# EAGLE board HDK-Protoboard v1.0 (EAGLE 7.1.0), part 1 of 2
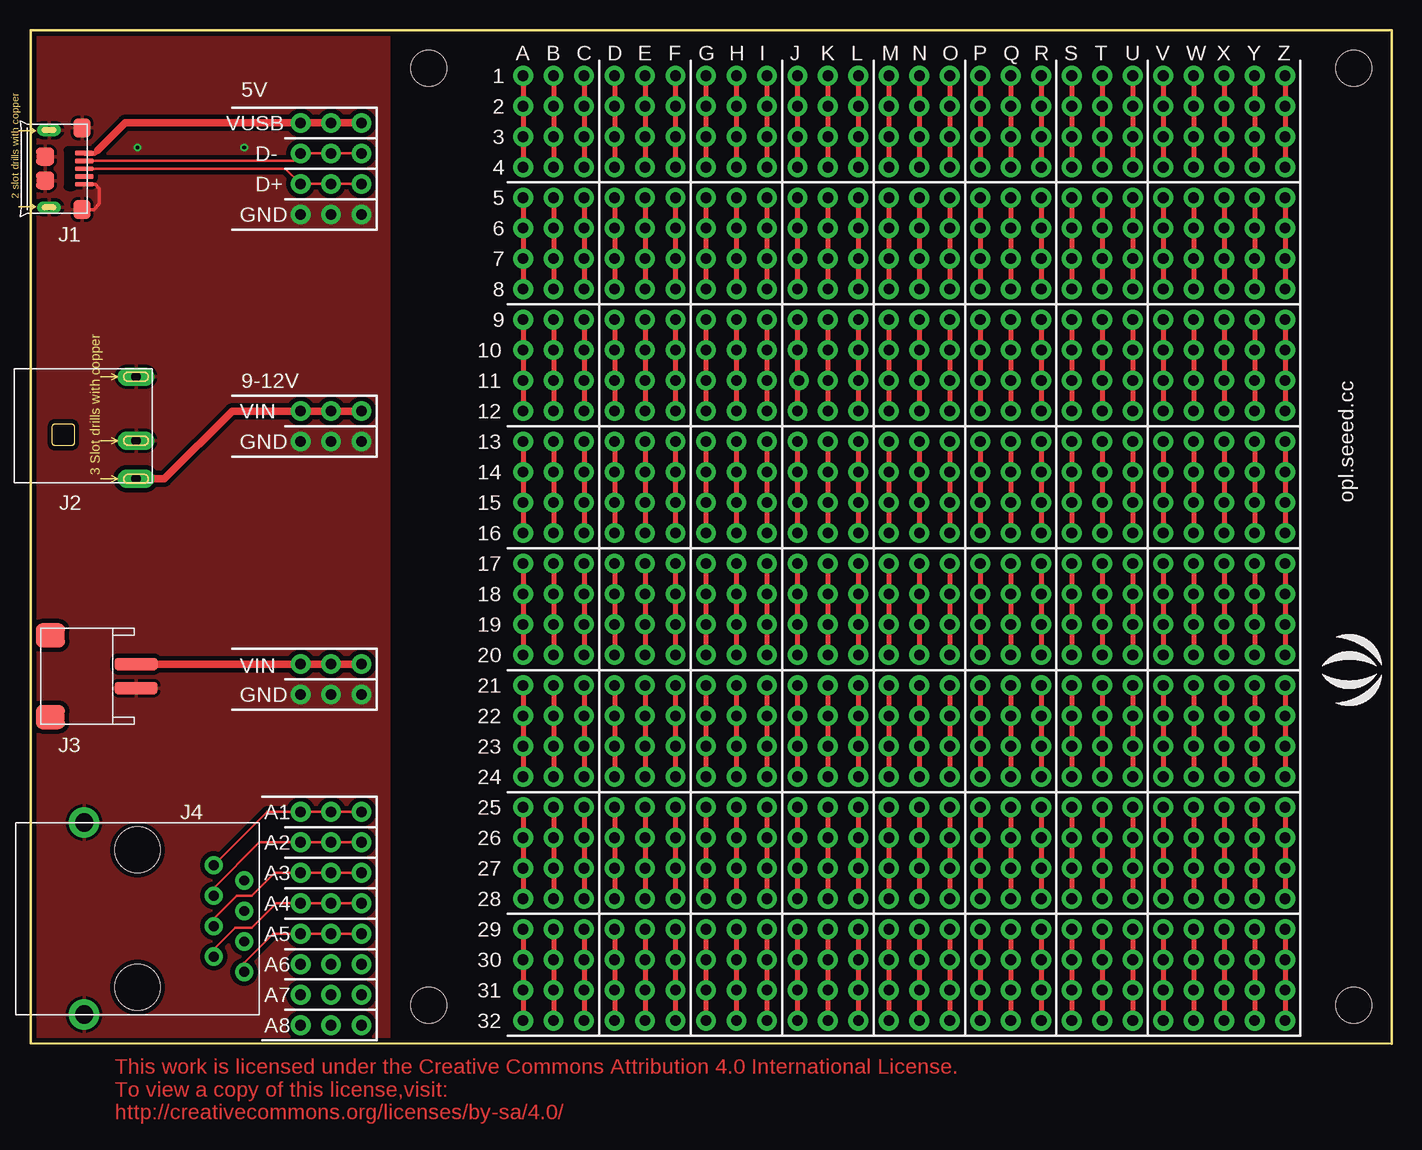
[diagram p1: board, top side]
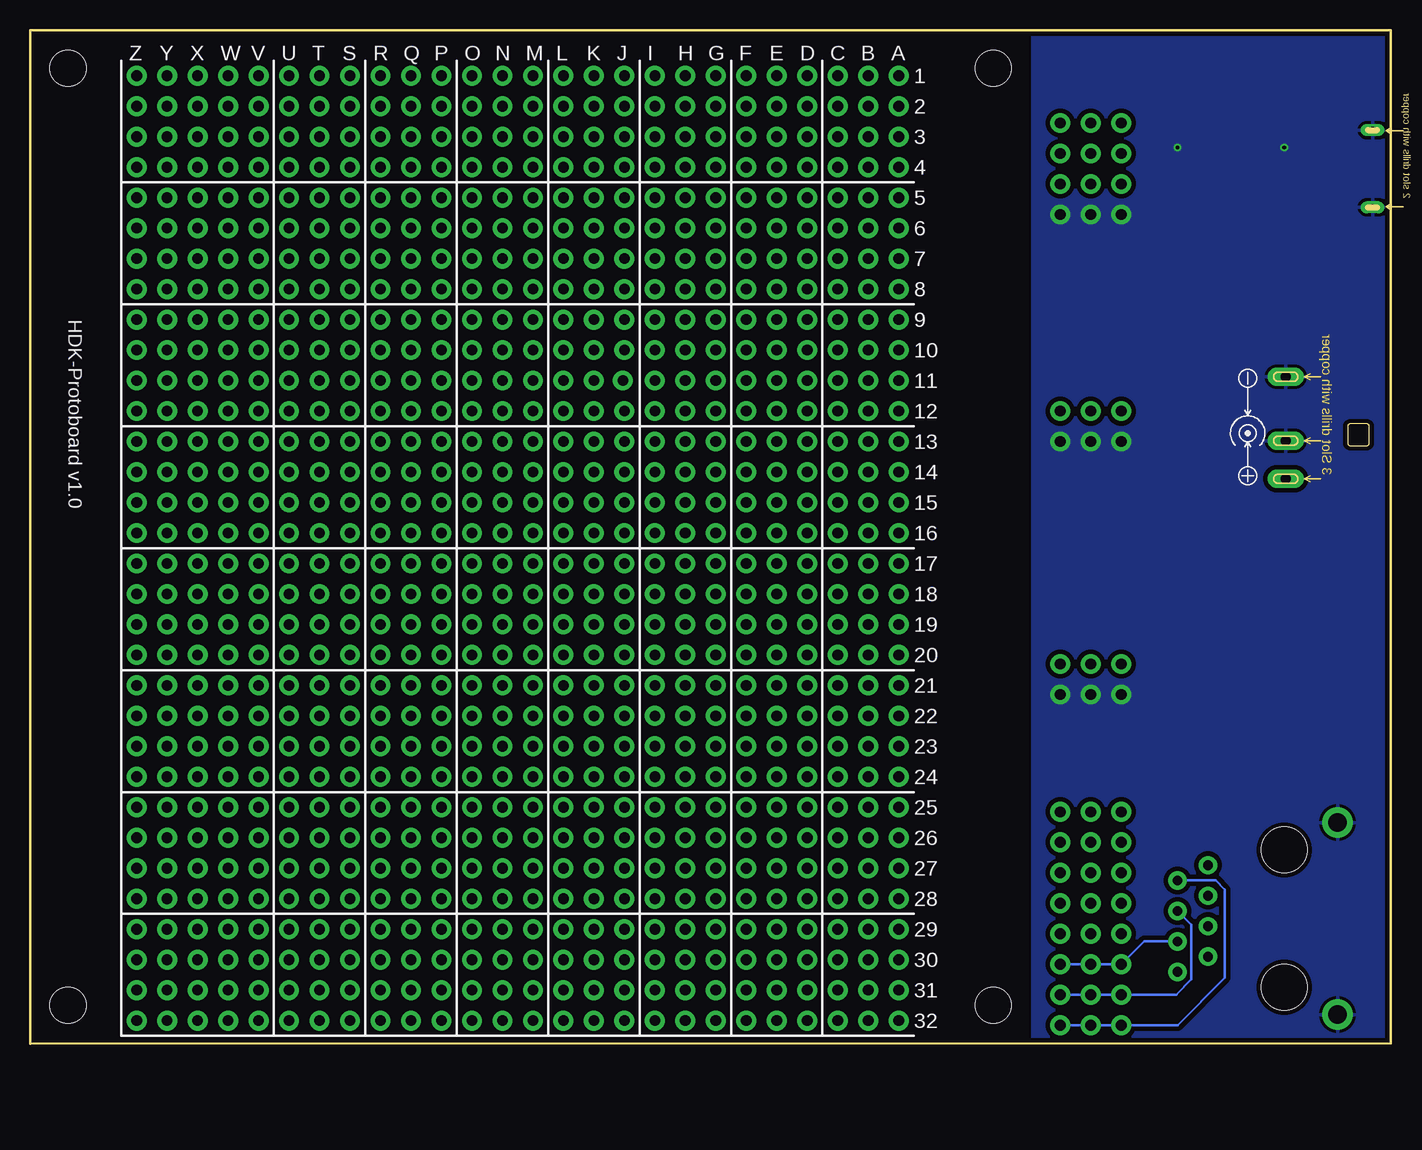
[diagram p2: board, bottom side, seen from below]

Size 113.41 x 84.46 mm. Coordinates in mm from the lower left corner, seen from the top.
Outline: 113.41,0 113.41,84.45 0,84.46 0,0.01 113.41,0
Copper layers (1*16): Top 0.035mm / dielectric 1.5mm / Bottom 0.035mm
Design rules "SeeedStudio_2layer_DRU_no_angle_20140221 *": minimum track width 1mil, minimum drill 12mil, track to track 6mil, track to pad 6mil, pad to pad 6mil, via to via 6mil, smd to smd 0mil, copper to edge 10mil, drill to drill 10mil, minimum pad ring 10mil, minimum via ring 6mil, stop-mask expansion 2mil, vias tented up to drill 25mil, thermal gap 10mil
Net classes: 2 gnd: width 0.305 mm, drill 0.559 mm, clearance 0.254 mm; 3 none3: width 0.203 mm, drill 0.305 mm, clearance 0.203 mm; 4 aref: width 0.406 mm, drill 0.61 mm, clearance 0.254 mm
Holes 3 mm at 110.24,81.28 110.24,3.18 33.15,81.28 33.15,3.18

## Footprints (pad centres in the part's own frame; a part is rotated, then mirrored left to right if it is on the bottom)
MICRO-USB5+4P-SMD-0.65-B-NO-HOLE = smd 0.381 x 1.524: 1 -1.3,-0.25; 2 -0.65,-0.25; 3 0,-0.25; 4 0.65,-0.25; 5 1.3,-0.25 | smd 1.6 x 1.397: S1 -3.4,-0.427; S6 3.4,-0.427 | drill 0.508 pad 1.016 long: S2 -3.226,-3.175; S5 3.226,-3.175 | smd 1.5 x 1.5: S3 -1,-3.5; S4 1,-3.5
DCJ3P-11.6X9.6X7.0MM = drill 0.813 pad 1.524 long: + 4.381,10.16; - -4.128,10.16; CDN 1.206,10.16
HW2-SMD-2.0-90D = smd 2 x 2.4: 3 3.4,-2.181; 4 -3.4,-2.181 | smd 1 x 3.6: + -1,4.953; - 1,4.953
RJ45-8P-20.4X16MM = drill 0.813 pad 1.524: A1 -2.54,5.08; A2 -2.54,2.54; A3 -2.54,0; A4 -2.54,-2.54; A5 0,-3.81; A6 0,-1.27; A7 0,1.27; A8 0,3.81 | drill 1.524 pad 2.54: GND0 -13.335,8.636; GND1 -13.335,-7.366 | hole 3.81: -8.89,-5.08; -8.89,6.35

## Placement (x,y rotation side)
FR1  [SEEEDSTUDIO-PCB-FRAME]  not placed on the board
J1  [MICRO-USB5+4P-SMD-0.65-B-NO-HOLE]  4.7,72.9 270 top
J2  [DCJ3P-11.6X9.6X7.0MM]  -1.4,51.44 270 top
J3  [HW2-SMD-2.0-90D]  3.81,30.61 270 top
J4  CONNECTER_RJ45_X1_DD  [RJ45-8P-20.4X16MM]  17.78,9.78 0 top
U$2  [SEEED-SILK-280*268MIL]  110.87,31.12 90 top

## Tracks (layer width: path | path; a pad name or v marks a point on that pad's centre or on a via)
A1  (via drill 0.89 pad 1.65)
  Top 0.203: J4.A1 19.69,19.31 v22.48,19.31 27.56,19.31
A2  (via drill 0.89 pad 1.65)
  Top 0.203: J4.A2 15.24,12.96 19.05,16.77 v22.48,16.77 27.56,16.77
A3  (via drill 0.89 pad 1.65)
  Top 0.203: J4.A3 15.24,10.42 17.14,12.32 18.41,12.32 20.32,14.23 v22.48,14.23 27.56,14.23
A4  (via drill 0.89 pad 1.65)
  Top 0.203: J4.A4 15.24,7.88 17.02,9.65 18.41,9.65 20.45,11.69 v22.48,11.69 27.56,11.69
A5  (via drill 0.89 pad 1.65)
  Top 0.203: J4.A5 17.78,6.73 20.19,9.15 v22.48,9.15 27.56,9.15
A6  (via drill 0.89 pad 1.65)
  Bottom 0.203: J4.A6 20.57,8.51 v22.48,6.61 27.56,6.61
A7  (via drill 0.89 pad 1.65)
  Bottom 0.203: J4.A7 16.64,9.91 16.64,5.34 17.91,4.07 v22.48,4.07 27.56,4.07
A8  (via drill 0.89 pad 1.65)
  Bottom 0.203: J4.A8 14.61,13.59 13.84,12.83 13.84,5.46 17.78,1.53 v22.48,1.53 27.56,1.53
D+2  (via drill 0.89 pad 1.65)
  Top 0.203: J1.3 21.21,72.9 v22.48,71.63 v25.02,71.63 v27.56,71.63
D-2  (via drill 0.89 pad 1.65)
  Top 0.203: J1.2 21.86,73.55 v22.48,74.17 v25.02,74.17 v27.56,74.17
GND  (via drill 0.3 pad 0.64, 0.89 pad 1.65)
  Top 0.305: J1.5 5.36,71.6 5.72,71.25 5.72,69.98 5.24,69.5 J1.S6
  other vias: 22.48,29.09 25.02,29.09 27.56,29.09 22.48,50.17 25.02,50.17 27.56,50.17 22.48,69.09 25.02,69.09 27.56,69.09 8.89,74.68 17.78,74.68
  pour Bottom (isolate 0.381, rank 6): -0.63,0 29.84,0 29.84,84.46 -0.63,84.46
  pour Top (isolate 0.381, rank 6): -0.63,0 29.84,0 29.84,84.46 -0.63,84.46
N$1  (via drill 0.89 pad 1.65)
  other vias: 41.02,1.91
N$2  (via drill 0.89 pad 1.65)
  other vias: 43.56,1.91
N$3  (via drill 0.89 pad 1.65)
  other vias: 46.1,1.91
N$4  (via drill 0.89 pad 1.65)
  other vias: 48.64,1.91
N$5  (via drill 0.89 pad 1.65)
  other vias: 51.18,1.91
N$6  (via drill 0.89 pad 1.65)
  other vias: 41.02,4.45
N$7  (via drill 0.89 pad 1.65)
  other vias: 43.56,4.45
N$8  (via drill 0.89 pad 1.65)
  other vias: 46.1,4.45
N$9  (via drill 0.89 pad 1.65)
  other vias: 48.64,4.45
N$10  (via drill 0.89 pad 1.65)
  other vias: 51.18,4.45
N$11  (via drill 0.89 pad 1.65)
  other vias: 53.72,1.91
N$12  (via drill 0.89 pad 1.65)
  other vias: 53.72,4.45
N$13  (via drill 0.89 pad 1.65)
  other vias: 56.26,4.45
N$14  (via drill 0.89 pad 1.65)
  other vias: 56.26,1.91
N$15  (via drill 0.89 pad 1.65)
  other vias: 58.8,4.45
N$16  (via drill 0.89 pad 1.65)
  other vias: 58.8,1.91
N$18  (via drill 0.89 pad 1.65)
  other vias: 61.34,4.45
N$19  (via drill 0.89 pad 1.65)
  other vias: 66.42,1.91
N$20  (via drill 0.89 pad 1.65)
  other vias: 68.96,4.45
N$21  (via drill 0.89 pad 1.65)
  other vias: 68.96,1.91
N$22  (via drill 0.89 pad 1.65)
  other vias: 71.5,4.45
N$23  (via drill 0.89 pad 1.65)
  other vias: 71.5,1.91
N$24  (via drill 0.89 pad 1.65)
  other vias: 74.04,4.45
N$25  (via drill 0.89 pad 1.65)
  other vias: 74.04,1.91
N$26  (via drill 0.89 pad 1.65)
  other vias: 76.58,4.45
N$27  (via drill 0.89 pad 1.65)
  other vias: 76.58,1.91
N$28  (via drill 0.89 pad 1.65)
  other vias: 79.12,4.45
N$29  (via drill 0.89 pad 1.65)
  other vias: 79.12,1.91
N$30  (via drill 0.89 pad 1.65)
  other vias: 81.66,4.45
N$31  (via drill 0.89 pad 1.65)
  other vias: 81.66,1.91
N$32  (via drill 0.89 pad 1.65)
  other vias: 84.2,4.45
N$33  (via drill 0.89 pad 1.65)
  other vias: 84.2,1.91
N$34  (via drill 0.89 pad 1.65)
  other vias: 86.74,1.91
N$35  (via drill 0.89 pad 1.65)
  other vias: 89.28,1.91
N$36  (via drill 0.89 pad 1.65)
  other vias: 91.82,1.91
N$37  (via drill 0.89 pad 1.65)
  other vias: 94.36,1.91
N$38  (via drill 0.89 pad 1.65)
  other vias: 96.9,1.91
N$39  (via drill 0.89 pad 1.65)
  other vias: 99.44,1.91
N$40  (via drill 0.89 pad 1.65)
  other vias: 101.98,1.91
N$41  (via drill 0.89 pad 1.65)
  other vias: 104.52,1.91
N$42  (via drill 0.89 pad 1.65)
  other vias: 86.74,4.45
N$43  (via drill 0.89 pad 1.65)
  other vias: 89.28,4.45
N$44  (via drill 0.89 pad 1.65)
  other vias: 91.82,4.45
N$45  (via drill 0.89 pad 1.65)
  other vias: 94.36,4.45
N$46  (via drill 0.89 pad 1.65)
  other vias: 96.9,4.45
N$47  (via drill 0.89 pad 1.65)
  other vias: 99.44,4.45
N$48  (via drill 0.89 pad 1.65)
  other vias: 101.98,4.45
N$49  (via drill 0.89 pad 1.65)
  other vias: 104.52,4.45
N$50  (via drill 0.89 pad 1.65)
  other vias: 41.02,6.99
N$51  (via drill 0.89 pad 1.65)
  other vias: 43.56,6.99
N$52  (via drill 0.89 pad 1.65)
  other vias: 46.1,6.99
N$53  (via drill 0.89 pad 1.65)
  other vias: 48.64,6.99
N$54  (via drill 0.89 pad 1.65)
  other vias: 51.18,6.99
N$55  (via drill 0.89 pad 1.65)
  Top 0.406: v41.02,9.53 41.02,1.91
N$56  (via drill 0.89 pad 1.65)
  other vias: 43.56,9.53
N$57  (via drill 0.89 pad 1.65)
  other vias: 46.1,9.53
N$58  (via drill 0.89 pad 1.65)
  other vias: 48.64,9.53
N$59  (via drill 0.89 pad 1.65)
  other vias: 51.18,9.53
N$60  (via drill 0.89 pad 1.65)
  other vias: 53.72,6.99
N$61  (via drill 0.89 pad 1.65)
  other vias: 53.72,9.53
N$62  (via drill 0.89 pad 1.65)
  other vias: 56.26,9.53
N$63  (via drill 0.89 pad 1.65)
  other vias: 56.26,6.99
N$64  (via drill 0.89 pad 1.65)
  other vias: 58.8,9.53
N$65  (via drill 0.89 pad 1.65)
  other vias: 58.8,6.99
N$67  (via drill 0.89 pad 1.65)
  other vias: 61.34,9.53
N$68  (via drill 0.89 pad 1.65)
  other vias: 66.42,6.99
N$69  (via drill 0.89 pad 1.65)
  other vias: 68.96,9.53
N$70  (via drill 0.89 pad 1.65)
  other vias: 68.96,6.99
N$71  (via drill 0.89 pad 1.65)
  other vias: 71.5,9.53
N$72  (via drill 0.89 pad 1.65)
  other vias: 71.5,6.99
N$73  (via drill 0.89 pad 1.65)
  other vias: 74.04,9.53
N$74  (via drill 0.89 pad 1.65)
  other vias: 74.04,6.99
N$75  (via drill 0.89 pad 1.65)
  other vias: 76.58,9.53
N$76  (via drill 0.89 pad 1.65)
  other vias: 76.58,6.99
N$77  (via drill 0.89 pad 1.65)
  other vias: 79.12,9.53
N$78  (via drill 0.89 pad 1.65)
  other vias: 79.12,6.99
N$79  (via drill 0.89 pad 1.65)
  other vias: 81.66,9.53
N$80  (via drill 0.89 pad 1.65)
  other vias: 81.66,6.99
N$81  (via drill 0.89 pad 1.65)
  other vias: 84.2,9.53
N$82  (via drill 0.89 pad 1.65)
  other vias: 84.2,6.99
N$83  (via drill 0.89 pad 1.65)
  other vias: 86.74,6.99
N$84  (via drill 0.89 pad 1.65)
  other vias: 89.28,6.99
N$85  (via drill 0.89 pad 1.65)
  other vias: 91.82,6.99
N$86  (via drill 0.89 pad 1.65)
  other vias: 94.36,6.99
N$87  (via drill 0.89 pad 1.65)
  other vias: 96.9,6.99
N$88  (via drill 0.89 pad 1.65)
  other vias: 99.44,6.99
N$89  (via drill 0.89 pad 1.65)
  other vias: 101.98,6.99
N$90  (via drill 0.89 pad 1.65)
  other vias: 104.52,6.99
N$91  (via drill 0.89 pad 1.65)
  other vias: 86.74,9.53
N$92  (via drill 0.89 pad 1.65)
  other vias: 89.28,9.53
N$93  (via drill 0.89 pad 1.65)
  other vias: 91.82,9.53
N$94  (via drill 0.89 pad 1.65)
  other vias: 94.36,9.53
N$95  (via drill 0.89 pad 1.65)
  other vias: 96.9,9.53
N$96  (via drill 0.89 pad 1.65)
  other vias: 99.44,9.53
N$97  (via drill 0.89 pad 1.65)
  other vias: 101.98,9.53
N$98  (via drill 0.89 pad 1.65)
  other vias: 104.52,9.53
N$99  (via drill 0.89 pad 1.65)
  other vias: 41.02,12.07
N$100  (via drill 0.89 pad 1.65)
  other vias: 43.56,12.07
N$101  (via drill 0.89 pad 1.65)
  other vias: 46.1,12.07
N$102  (via drill 0.89 pad 1.65)
  other vias: 48.64,12.07
N$103  (via drill 0.89 pad 1.65)
  other vias: 51.18,12.07
N$104  (via drill 0.89 pad 1.65)
  other vias: 41.02,14.61
N$105  (via drill 0.89 pad 1.65)
  other vias: 43.56,14.61
N$106  (via drill 0.89 pad 1.65)
  other vias: 46.1,14.61
N$107  (via drill 0.89 pad 1.65)
  other vias: 48.64,14.61
N$108  (via drill 0.89 pad 1.65)
  other vias: 51.18,14.61
N$109  (via drill 0.89 pad 1.65)
  other vias: 53.72,12.07
N$110  (via drill 0.89 pad 1.65)
  other vias: 53.72,14.61
N$111  (via drill 0.89 pad 1.65)
  other vias: 56.26,14.61
N$112  (via drill 0.89 pad 1.65)
  other vias: 56.26,12.07
N$113  (via drill 0.89 pad 1.65)
  other vias: 58.8,14.61
N$114  (via drill 0.89 pad 1.65)
  other vias: 58.8,12.07
N$116  (via drill 0.89 pad 1.65)
  other vias: 61.34,14.61
N$117  (via drill 0.89 pad 1.65)
  other vias: 66.42,12.07
N$118  (via drill 0.89 pad 1.65)
  other vias: 68.96,14.61
N$119  (via drill 0.89 pad 1.65)
  other vias: 68.96,12.07
N$120  (via drill 0.89 pad 1.65)
  other vias: 71.5,14.61
N$121  (via drill 0.89 pad 1.65)
  other vias: 71.5,12.07
N$122  (via drill 0.89 pad 1.65)
  other vias: 74.04,14.61
N$123  (via drill 0.89 pad 1.65)
  other vias: 74.04,12.07
N$124  (via drill 0.89 pad 1.65)
  other vias: 76.58,14.61
N$125  (via drill 0.89 pad 1.65)
  other vias: 76.58,12.07
N$126  (via drill 0.89 pad 1.65)
  other vias: 79.12,14.61
N$127  (via drill 0.89 pad 1.65)
  other vias: 79.12,12.07
N$128  (via drill 0.89 pad 1.65)
  other vias: 81.66,14.61
N$129  (via drill 0.89 pad 1.65)
  other vias: 81.66,12.07
N$130  (via drill 0.89 pad 1.65)
  other vias: 84.2,14.61
N$131  (via drill 0.89 pad 1.65)
  other vias: 84.2,12.07
N$132  (via drill 0.89 pad 1.65)
  other vias: 86.74,12.07
N$133  (via drill 0.89 pad 1.65)
  other vias: 89.28,12.07
N$134  (via drill 0.89 pad 1.65)
  other vias: 91.82,12.07
N$135  (via drill 0.89 pad 1.65)
  other vias: 94.36,12.07
N$136  (via drill 0.89 pad 1.65)
  other vias: 96.9,12.07
N$137  (via drill 0.89 pad 1.65)
  other vias: 99.44,12.07
N$138  (via drill 0.89 pad 1.65)
  other vias: 101.98,12.07
N$139  (via drill 0.89 pad 1.65)
  other vias: 104.52,12.07
N$140  (via drill 0.89 pad 1.65)
  other vias: 86.74,14.61
N$141  (via drill 0.89 pad 1.65)
  other vias: 89.28,14.61
N$142  (via drill 0.89 pad 1.65)
  other vias: 91.82,14.61
N$143  (via drill 0.89 pad 1.65)
  other vias: 94.36,14.61
N$144  (via drill 0.89 pad 1.65)
  other vias: 96.9,14.61
N$145  (via drill 0.89 pad 1.65)
  other vias: 99.44,14.61
N$146  (via drill 0.89 pad 1.65)
  other vias: 101.98,14.61
N$147  (via drill 0.89 pad 1.65)
  other vias: 104.52,14.61
N$148  (via drill 0.89 pad 1.65)
  other vias: 41.02,17.15
N$149  (via drill 0.89 pad 1.65)
  other vias: 43.56,17.15
N$150  (via drill 0.89 pad 1.65)
  other vias: 46.1,17.15
N$151  (via drill 0.89 pad 1.65)
  other vias: 48.64,17.15
N$152  (via drill 0.89 pad 1.65)
  other vias: 51.18,17.15
N$153  (via drill 0.89 pad 1.65)
  Top 0.406: v41.02,19.69 41.02,12.07
N$154  (via drill 0.89 pad 1.65)
  other vias: 43.56,19.69
N$155  (via drill 0.89 pad 1.65)
  other vias: 46.1,19.69
N$156  (via drill 0.89 pad 1.65)
  other vias: 48.64,19.69
N$157  (via drill 0.89 pad 1.65)
  other vias: 51.18,19.69
N$158  (via drill 0.89 pad 1.65)
  other vias: 53.72,17.15
N$159  (via drill 0.89 pad 1.65)
  other vias: 53.72,19.69
N$160  (via drill 0.89 pad 1.65)
  other vias: 56.26,19.69
N$161  (via drill 0.89 pad 1.65)
  other vias: 56.26,17.15
N$162  (via drill 0.89 pad 1.65)
  other vias: 58.8,19.69
N$163  (via drill 0.89 pad 1.65)
  other vias: 58.8,17.15
N$165  (via drill 0.89 pad 1.65)
  other vias: 61.34,19.69
N$166  (via drill 0.89 pad 1.65)
  other vias: 66.42,17.15
N$167  (via drill 0.89 pad 1.65)
  other vias: 68.96,19.69
N$168  (via drill 0.89 pad 1.65)
  other vias: 68.96,17.15
N$169  (via drill 0.89 pad 1.65)
  other vias: 71.5,19.69
N$170  (via drill 0.89 pad 1.65)
  other vias: 71.5,17.15
N$171  (via drill 0.89 pad 1.65)
  other vias: 74.04,19.69
N$172  (via drill 0.89 pad 1.65)
  other vias: 74.04,17.15
N$173  (via drill 0.89 pad 1.65)
  other vias: 76.58,19.69
N$174  (via drill 0.89 pad 1.65)
  other vias: 76.58,17.15
N$175  (via drill 0.89 pad 1.65)
  other vias: 79.12,19.69
N$176  (via drill 0.89 pad 1.65)
  other vias: 79.12,17.15
N$177  (via drill 0.89 pad 1.65)
  other vias: 81.66,19.69
N$178  (via drill 0.89 pad 1.65)
  other vias: 81.66,17.15
N$179  (via drill 0.89 pad 1.65)
  other vias: 84.2,19.69
N$180  (via drill 0.89 pad 1.65)
  other vias: 84.2,17.15
N$181  (via drill 0.89 pad 1.65)
  other vias: 86.74,17.15
N$182  (via drill 0.89 pad 1.65)
  other vias: 89.28,17.15
N$183  (via drill 0.89 pad 1.65)
  other vias: 91.82,17.15
N$184  (via drill 0.89 pad 1.65)
  other vias: 94.36,17.15
N$185  (via drill 0.89 pad 1.65)
  other vias: 96.9,17.15
N$186  (via drill 0.89 pad 1.65)
  other vias: 99.44,17.15
N$187  (via drill 0.89 pad 1.65)
  other vias: 101.98,17.15
N$188  (via drill 0.89 pad 1.65)
  other vias: 104.52,17.15
N$189  (via drill 0.89 pad 1.65)
  other vias: 86.74,19.69
N$190  (via drill 0.89 pad 1.65)
  other vias: 89.28,19.69
N$191  (via drill 0.89 pad 1.65)
  other vias: 91.82,19.69
N$192  (via drill 0.89 pad 1.65)
  other vias: 94.36,19.69
N$193  (via drill 0.89 pad 1.65)
  other vias: 96.9,19.69
N$194  (via drill 0.89 pad 1.65)
  other vias: 99.44,19.69
N$195  (via drill 0.89 pad 1.65)
  other vias: 101.98,19.69
N$196  (via drill 0.89 pad 1.65)
  other vias: 104.52,19.69
N$197  (via drill 0.89 pad 1.65)
  other vias: 41.02,22.23
N$198  (via drill 0.89 pad 1.65)
  other vias: 43.56,22.23
N$199  (via drill 0.89 pad 1.65)
  other vias: 46.1,22.23
N$200  (via drill 0.89 pad 1.65)
  other vias: 48.64,22.23
N$201  (via drill 0.89 pad 1.65)
  other vias: 51.18,22.23
N$202  (via drill 0.89 pad 1.65)
  other vias: 41.02,24.77
N$203  (via drill 0.89 pad 1.65)
  other vias: 43.56,24.77
N$204  (via drill 0.89 pad 1.65)
  other vias: 46.1,24.77
N$205  (via drill 0.89 pad 1.65)
  other vias: 48.64,24.77
N$206  (via drill 0.89 pad 1.65)
  other vias: 51.18,24.77
N$207  (via drill 0.89 pad 1.65)
  other vias: 53.72,22.23
N$208  (via drill 0.89 pad 1.65)
  other vias: 53.72,24.77
N$209  (via drill 0.89 pad 1.65)
  other vias: 56.26,24.77
N$210  (via drill 0.89 pad 1.65)
  other vias: 56.26,22.23
N$211  (via drill 0.89 pad 1.65)
  other vias: 58.8,24.77
N$212  (via drill 0.89 pad 1.65)
  other vias: 58.8,22.23
N$214  (via drill 0.89 pad 1.65)
  other vias: 61.34,24.77
N$215  (via drill 0.89 pad 1.65)
  other vias: 66.42,22.23
N$216  (via drill 0.89 pad 1.65)
  other vias: 68.96,24.77
N$217  (via drill 0.89 pad 1.65)
  other vias: 68.96,22.23
N$218  (via drill 0.89 pad 1.65)
  other vias: 71.5,24.77
N$219  (via drill 0.89 pad 1.65)
  other vias: 71.5,22.23
N$220  (via drill 0.89 pad 1.65)
  other vias: 74.04,24.77
N$221  (via drill 0.89 pad 1.65)
  other vias: 74.04,22.23
N$222  (via drill 0.89 pad 1.65)
  other vias: 76.58,24.77
N$223  (via drill 0.89 pad 1.65)
  other vias: 76.58,22.23
N$224  (via drill 0.89 pad 1.65)
  other vias: 79.12,24.77
N$225  (via drill 0.89 pad 1.65)
  other vias: 79.12,22.23
N$226  (via drill 0.89 pad 1.65)
  other vias: 81.66,24.77
N$227  (via drill 0.89 pad 1.65)
  other vias: 81.66,22.23
N$228  (via drill 0.89 pad 1.65)
  other vias: 84.2,24.77
N$229  (via drill 0.89 pad 1.65)
  other vias: 84.2,22.23
N$230  (via drill 0.89 pad 1.65)
  other vias: 86.74,22.23
N$231  (via drill 0.89 pad 1.65)
  other vias: 89.28,22.23
N$232  (via drill 0.89 pad 1.65)
  other vias: 91.82,22.23
N$233  (via drill 0.89 pad 1.65)
  other vias: 94.36,22.23
N$234  (via drill 0.89 pad 1.65)
  other vias: 96.9,22.23
N$235  (via drill 0.89 pad 1.65)
  other vias: 99.44,22.23
N$236  (via drill 0.89 pad 1.65)
  other vias: 101.98,22.23
N$237  (via drill 0.89 pad 1.65)
  other vias: 104.52,22.23
N$238  (via drill 0.89 pad 1.65)
  other vias: 86.74,24.77
N$239  (via drill 0.89 pad 1.65)
  other vias: 89.28,24.77
N$240  (via drill 0.89 pad 1.65)
  other vias: 91.82,24.77
N$241  (via drill 0.89 pad 1.65)
  other vias: 94.36,24.77
N$242  (via drill 0.89 pad 1.65)
  other vias: 96.9,24.77
N$243  (via drill 0.89 pad 1.65)
  other vias: 99.44,24.77
N$244  (via drill 0.89 pad 1.65)
  other vias: 101.98,24.77
N$245  (via drill 0.89 pad 1.65)
  other vias: 104.52,24.77
N$246  (via drill 0.89 pad 1.65)
  other vias: 41.02,27.31
N$247  (via drill 0.89 pad 1.65)
  other vias: 43.56,27.31
N$248  (via drill 0.89 pad 1.65)
  other vias: 46.1,27.31
N$249  (via drill 0.89 pad 1.65)
  other vias: 48.64,27.31
N$250  (via drill 0.89 pad 1.65)
  other vias: 51.18,27.31
N$251  (via drill 0.89 pad 1.65)
  Top 0.406: v41.02,29.85 41.02,22.23
N$252  (via drill 0.89 pad 1.65)
  other vias: 43.56,29.85
N$253  (via drill 0.89 pad 1.65)
  other vias: 46.1,29.85
N$254  (via drill 0.89 pad 1.65)
  other vias: 48.64,29.85
N$255  (via drill 0.89 pad 1.65)
  other vias: 51.18,29.85
N$256  (via drill 0.89 pad 1.65)
  other vias: 53.72,27.31
N$257  (via drill 0.89 pad 1.65)
  other vias: 53.72,29.85
N$258  (via drill 0.89 pad 1.65)
  other vias: 56.26,29.85
N$259  (via drill 0.89 pad 1.65)
  other vias: 56.26,27.31
N$260  (via drill 0.89 pad 1.65)
  other vias: 58.8,29.85
N$261  (via drill 0.89 pad 1.65)
  other vias: 58.8,27.31
N$263  (via drill 0.89 pad 1.65)
  other vias: 61.34,29.85
N$264  (via drill 0.89 pad 1.65)
  other vias: 66.42,27.31
N$265  (via drill 0.89 pad 1.65)
  other vias: 68.96,29.85
N$266  (via drill 0.89 pad 1.65)
  other vias: 68.96,27.31
N$267  (via drill 0.89 pad 1.65)
  other vias: 71.5,29.85
N$268  (via drill 0.89 pad 1.65)
  other vias: 71.5,27.31
N$269  (via drill 0.89 pad 1.65)
  other vias: 74.04,29.85
N$270  (via drill 0.89 pad 1.65)
  other vias: 74.04,27.31
N$271  (via drill 0.89 pad 1.65)
  other vias: 76.58,29.85
N$272  (via drill 0.89 pad 1.65)
  other vias: 76.58,27.31
N$273  (via drill 0.89 pad 1.65)
  other vias: 79.12,29.85
N$274  (via drill 0.89 pad 1.65)
  other vias: 79.12,27.31
N$275  (via drill 0.89 pad 1.65)
  other vias: 81.66,29.85
N$276  (via drill 0.89 pad 1.65)
  other vias: 81.66,27.31
N$277  (via drill 0.89 pad 1.65)
  other vias: 84.2,29.85
N$278  (via drill 0.89 pad 1.65)
  other vias: 84.2,27.31
N$279  (via drill 0.89 pad 1.65)
  other vias: 86.74,27.31
N$280  (via drill 0.89 pad 1.65)
  other vias: 89.28,27.31
N$281  (via drill 0.89 pad 1.65)
  other vias: 91.82,27.31
N$282  (via drill 0.89 pad 1.65)
  other vias: 94.36,27.31
N$283  (via drill 0.89 pad 1.65)
  other vias: 96.9,27.31
N$284  (via drill 0.89 pad 1.65)
  other vias: 99.44,27.31
N$285  (via drill 0.89 pad 1.65)
  other vias: 101.98,27.31
N$286  (via drill 0.89 pad 1.65)
  other vias: 104.52,27.31
N$287  (via drill 0.89 pad 1.65)
  other vias: 86.74,29.85
N$288  (via drill 0.89 pad 1.65)
  other vias: 89.28,29.85
N$289  (via drill 0.89 pad 1.65)
  other vias: 91.82,29.85
N$290  (via drill 0.89 pad 1.65)
  other vias: 94.36,29.85
N$291  (via drill 0.89 pad 1.65)
  other vias: 96.9,29.85
N$292  (via drill 0.89 pad 1.65)
  other vias: 99.44,29.85
N$293  (via drill 0.89 pad 1.65)
  other vias: 101.98,29.85
N$294  (via drill 0.89 pad 1.65)
  other vias: 104.52,29.85
N$295  (via drill 0.89 pad 1.65)
  other vias: 41.02,32.39
N$296  (via drill 0.89 pad 1.65)
  other vias: 43.56,32.39
N$297  (via drill 0.89 pad 1.65)
  other vias: 46.1,32.39
N$298  (via drill 0.89 pad 1.65)
  other vias: 48.64,32.39
N$299  (via drill 0.89 pad 1.65)
  other vias: 51.18,32.39
N$300  (via drill 0.89 pad 1.65)
  other vias: 41.02,34.93
N$301  (via drill 0.89 pad 1.65)
  other vias: 43.56,34.93
N$302  (via drill 0.89 pad 1.65)
  other vias: 46.1,34.93
N$303  (via drill 0.89 pad 1.65)
  other vias: 48.64,34.93
N$304  (via drill 0.89 pad 1.65)
  other vias: 51.18,34.93
N$305  (via drill 0.89 pad 1.65)
  other vias: 53.72,32.39
N$306  (via drill 0.89 pad 1.65)
  other vias: 53.72,34.93
N$307  (via drill 0.89 pad 1.65)
  other vias: 56.26,34.93
N$308  (via drill 0.89 pad 1.65)
  other vias: 56.26,32.39
N$309  (via drill 0.89 pad 1.65)
  other vias: 58.8,34.93
N$310  (via drill 0.89 pad 1.65)
  other vias: 58.8,32.39
N$312  (via drill 0.89 pad 1.65)
  other vias: 61.34,34.93
N$313  (via drill 0.89 pad 1.65)
  other vias: 66.42,32.39
N$314  (via drill 0.89 pad 1.65)
  other vias: 68.96,34.93
N$315  (via drill 0.89 pad 1.65)
  other vias: 68.96,32.39
N$316  (via drill 0.89 pad 1.65)
  other vias: 71.5,34.93
N$317  (via drill 0.89 pad 1.65)
  other vias: 71.5,32.39
N$318  (via drill 0.89 pad 1.65)
  other vias: 74.04,34.93
N$319  (via drill 0.89 pad 1.65)
  other vias: 74.04,32.39
N$320  (via drill 0.89 pad 1.65)
  other vias: 76.58,34.93
N$321  (via drill 0.89 pad 1.65)
  other vias: 76.58,32.39
N$322  (via drill 0.89 pad 1.65)
  other vias: 79.12,34.93
N$323  (via drill 0.89 pad 1.65)
  other vias: 79.12,32.39
N$324  (via drill 0.89 pad 1.65)
  other vias: 81.66,34.93
N$325  (via drill 0.89 pad 1.65)
  other vias: 81.66,32.39
N$326  (via drill 0.89 pad 1.65)
  other vias: 84.2,34.93
N$327  (via drill 0.89 pad 1.65)
  other vias: 84.2,32.39
N$328  (via drill 0.89 pad 1.65)
  other vias: 86.74,32.39
N$329  (via drill 0.89 pad 1.65)
  other vias: 89.28,32.39
N$330  (via drill 0.89 pad 1.65)
  other vias: 91.82,32.39
N$331  (via drill 0.89 pad 1.65)
  other vias: 94.36,32.39
N$332  (via drill 0.89 pad 1.65)
  other vias: 96.9,32.39
N$333  (via drill 0.89 pad 1.65)
  other vias: 99.44,32.39
N$334  (via drill 0.89 pad 1.65)
  other vias: 101.98,32.39
N$335  (via drill 0.89 pad 1.65)
  other vias: 104.52,32.39
N$336  (via drill 0.89 pad 1.65)
  other vias: 86.74,34.93
N$337  (via drill 0.89 pad 1.65)
  other vias: 89.28,34.93
N$338  (via drill 0.89 pad 1.65)
  other vias: 91.82,34.93
N$339  (via drill 0.89 pad 1.65)
  other vias: 94.36,34.93
N$340  (via drill 0.89 pad 1.65)
  other vias: 96.9,34.93
N$341  (via drill 0.89 pad 1.65)
  other vias: 99.44,34.93
N$342  (via drill 0.89 pad 1.65)
  other vias: 101.98,34.93
N$343  (via drill 0.89 pad 1.65)
  other vias: 104.52,34.93
N$344  (via drill 0.89 pad 1.65)
  other vias: 41.02,37.47
N$345  (via drill 0.89 pad 1.65)
  other vias: 43.56,37.47
N$346  (via drill 0.89 pad 1.65)
  other vias: 46.1,37.47
N$347  (via drill 0.89 pad 1.65)
  other vias: 48.64,37.47
N$348  (via drill 0.89 pad 1.65)
  other vias: 51.18,37.47
N$349  (via drill 0.89 pad 1.65)
  Top 0.406: v41.02,40.01 41.02,32.39
N$350  (via drill 0.89 pad 1.65)
  other vias: 43.56,40.01
N$351  (via drill 0.89 pad 1.65)
  other vias: 46.1,40.01
N$352  (via drill 0.89 pad 1.65)
  other vias: 48.64,40.01
N$353  (via drill 0.89 pad 1.65)
  other vias: 51.18,40.01
N$354  (via drill 0.89 pad 1.65)
  other vias: 53.72,37.47
N$355  (via drill 0.89 pad 1.65)
  other vias: 53.72,40.01
N$356  (via drill 0.89 pad 1.65)
  other vias: 56.26,40.01
N$357  (via drill 0.89 pad 1.65)
  other vias: 56.26,37.47
N$358  (via drill 0.89 pad 1.65)
  other vias: 58.8,40.01
N$359  (via drill 0.89 pad 1.65)
  other vias: 58.8,37.47
N$360  (via drill 0.89 pad 1.65)
  other vias: 61.34,37.47
N$361  (via drill 0.89 pad 1.65)
  other vias: 61.34,40.01
N$362  (via drill 0.89 pad 1.65)
  other vias: 66.42,37.47
N$363  (via drill 0.89 pad 1.65)
  other vias: 68.96,40.01
N$364  (via drill 0.89 pad 1.65)
  other vias: 68.96,37.47
N$365  (via drill 0.89 pad 1.65)
  other vias: 71.5,40.01
N$366  (via drill 0.89 pad 1.65)
  other vias: 71.5,37.47
N$367  (via drill 0.89 pad 1.65)
  other vias: 74.04,40.01
N$368  (via drill 0.89 pad 1.65)
  other vias: 74.04,37.47
N$369  (via drill 0.89 pad 1.65)
  other vias: 76.58,40.01
N$370  (via drill 0.89 pad 1.65)
  other vias: 76.58,37.47
N$371  (via drill 0.89 pad 1.65)
  other vias: 79.12,40.01
N$372  (via drill 0.89 pad 1.65)
  other vias: 79.12,37.47
N$373  (via drill 0.89 pad 1.65)
  other vias: 81.66,40.01
N$374  (via drill 0.89 pad 1.65)
  other vias: 81.66,37.47
N$375  (via drill 0.89 pad 1.65)
  other vias: 84.2,40.01
N$376  (via drill 0.89 pad 1.65)
  other vias: 84.2,37.47
N$377  (via drill 0.89 pad 1.65)
  other vias: 86.74,37.47
N$378  (via drill 0.89 pad 1.65)
  other vias: 89.28,37.47
N$379  (via drill 0.89 pad 1.65)
  other vias: 91.82,37.47
N$380  (via drill 0.89 pad 1.65)
  other vias: 94.36,37.47
N$381  (via drill 0.89 pad 1.65)
  other vias: 96.9,37.47
N$382  (via drill 0.89 pad 1.65)
  other vias: 99.44,37.47
N$383  (via drill 0.89 pad 1.65)
  other vias: 101.98,37.47
N$384  (via drill 0.89 pad 1.65)
  other vias: 104.52,37.47
N$385  (via drill 0.89 pad 1.65)
  other vias: 86.74,40.01
N$386  (via drill 0.89 pad 1.65)
  other vias: 89.28,40.01
N$387  (via drill 0.89 pad 1.65)
  other vias: 91.82,40.01
N$388  (via drill 0.89 pad 1.65)
  other vias: 94.36,40.01
N$389  (via drill 0.89 pad 1.65)
  other vias: 96.9,40.01
N$390  (via drill 0.89 pad 1.65)
  other vias: 99.44,40.01
N$391  (via drill 0.89 pad 1.65)
  other vias: 101.98,40.01
N$392  (via drill 0.89 pad 1.65)
  other vias: 104.52,40.01
N$393  (via drill 0.89 pad 1.65)
  other vias: 41.02,42.55
N$394  (via drill 0.89 pad 1.65)
  other vias: 43.56,42.55
N$395  (via drill 0.89 pad 1.65)
  other vias: 46.1,42.55
N$396  (via drill 0.89 pad 1.65)
  other vias: 48.64,42.55
N$397  (via drill 0.89 pad 1.65)
  other vias: 51.18,42.55
N$398  (via drill 0.89 pad 1.65)
  other vias: 41.02,45.09
N$399  (via drill 0.89 pad 1.65)
  other vias: 43.56,45.09
N$400  (via drill 0.89 pad 1.65)
  other vias: 46.1,45.09
N$401  (via drill 0.89 pad 1.65)
  other vias: 48.64,45.09
N$402  (via drill 0.89 pad 1.65)
  other vias: 51.18,45.09
N$403  (via drill 0.89 pad 1.65)
  other vias: 53.72,42.55
N$404  (via drill 0.89 pad 1.65)
  other vias: 53.72,45.09
N$405  (via drill 0.89 pad 1.65)
  other vias: 56.26,45.09
N$406  (via drill 0.89 pad 1.65)
  other vias: 56.26,42.55
N$407  (via drill 0.89 pad 1.65)
  other vias: 58.8,45.09
N$408  (via drill 0.89 pad 1.65)
  other vias: 58.8,42.55
N$409  (via drill 0.89 pad 1.65)
  other vias: 63.88,80.65
N$410  (via drill 0.89 pad 1.65)
  other vias: 61.34,45.09
N$411  (via drill 0.89 pad 1.65)
  other vias: 66.42,42.55
N$412  (via drill 0.89 pad 1.65)
  other vias: 68.96,45.09
N$413  (via drill 0.89 pad 1.65)
  other vias: 68.96,42.55
N$414  (via drill 0.89 pad 1.65)
  other vias: 71.5,45.09
N$415  (via drill 0.89 pad 1.65)
  other vias: 71.5,42.55
N$416  (via drill 0.89 pad 1.65)
  other vias: 74.04,45.09
N$417  (via drill 0.89 pad 1.65)
  other vias: 74.04,42.55
N$418  (via drill 0.89 pad 1.65)
  other vias: 76.58,45.09
N$419  (via drill 0.89 pad 1.65)
  other vias: 76.58,42.55
N$420  (via drill 0.89 pad 1.65)
  other vias: 79.12,45.09
N$421  (via drill 0.89 pad 1.65)
  other vias: 79.12,42.55
N$422  (via drill 0.89 pad 1.65)
  other vias: 81.66,45.09
N$423  (via drill 0.89 pad 1.65)
  other vias: 81.66,42.55
N$424  (via drill 0.89 pad 1.65)
  other vias: 84.2,45.09
N$425  (via drill 0.89 pad 1.65)
  other vias: 84.2,42.55
N$426  (via drill 0.89 pad 1.65)
  other vias: 86.74,42.55
N$427  (via drill 0.89 pad 1.65)
  other vias: 89.28,42.55
N$428  (via drill 0.89 pad 1.65)
  other vias: 91.82,42.55
N$429  (via drill 0.89 pad 1.65)
  other vias: 94.36,42.55
N$430  (via drill 0.89 pad 1.65)
  other vias: 96.9,42.55
N$431  (via drill 0.89 pad 1.65)
  other vias: 99.44,42.55
N$432  (via drill 0.89 pad 1.65)
  other vias: 101.98,42.55
N$433  (via drill 0.89 pad 1.65)
  other vias: 104.52,42.55
N$434  (via drill 0.89 pad 1.65)
  other vias: 86.74,45.09
N$435  (via drill 0.89 pad 1.65)
  other vias: 89.28,45.09
N$436  (via drill 0.89 pad 1.65)
  other vias: 91.82,45.09
N$437  (via drill 0.89 pad 1.65)
  other vias: 94.36,45.09
N$438  (via drill 0.89 pad 1.65)
  other vias: 96.9,45.09
N$439  (via drill 0.89 pad 1.65)
  other vias: 99.44,45.09
N$440  (via drill 0.89 pad 1.65)
  other vias: 101.98,45.09
N$441  (via drill 0.89 pad 1.65)
  other vias: 104.52,45.09
N$442  (via drill 0.89 pad 1.65)
  other vias: 41.02,47.63
N$443  (via drill 0.89 pad 1.65)
  other vias: 43.56,47.63
N$444  (via drill 0.89 pad 1.65)
  other vias: 46.1,47.63
N$445  (via drill 0.89 pad 1.65)
  other vias: 48.64,47.63
N$446  (via drill 0.89 pad 1.65)
  other vias: 51.18,47.63
N$447  (via drill 0.89 pad 1.65)
  Top 0.406: v41.02,50.17 41.02,42.55
N$448  (via drill 0.89 pad 1.65)
  other vias: 43.56,50.17
N$449  (via drill 0.89 pad 1.65)
  other vias: 46.1,50.17
N$450  (via drill 0.89 pad 1.65)
  other vias: 48.64,50.17
N$451  (via drill 0.89 pad 1.65)
  other vias: 51.18,50.17
N$452  (via drill 0.89 pad 1.65)
  other vias: 53.72,47.63
N$453  (via drill 0.89 pad 1.65)
  other vias: 53.72,50.17
N$454  (via drill 0.89 pad 1.65)
  other vias: 56.26,50.17
N$455  (via drill 0.89 pad 1.65)
  other vias: 56.26,47.63
N$456  (via drill 0.89 pad 1.65)
  other vias: 58.8,50.17
N$457  (via drill 0.89 pad 1.65)
  other vias: 58.8,47.63
N$458  (via drill 0.89 pad 1.65)
  other vias: 66.42,80.65
N$459  (via drill 0.89 pad 1.65)
  other vias: 61.34,50.17
N$460  (via drill 0.89 pad 1.65)
  other vias: 66.42,47.63
N$461  (via drill 0.89 pad 1.65)
  other vias: 68.96,50.17
N$462  (via drill 0.89 pad 1.65)
  other vias: 68.96,47.63
N$463  (via drill 0.89 pad 1.65)
  other vias: 71.5,50.17
N$464  (via drill 0.89 pad 1.65)
  other vias: 71.5,47.63
N$465  (via drill 0.89 pad 1.65)
  other vias: 74.04,50.17
N$466  (via drill 0.89 pad 1.65)
  other vias: 74.04,47.63
N$467  (via drill 0.89 pad 1.65)
  other vias: 76.58,50.17
N$468  (via drill 0.89 pad 1.65)
  other vias: 76.58,47.63
N$469  (via drill 0.89 pad 1.65)
  other vias: 79.12,50.17
N$470  (via drill 0.89 pad 1.65)
  other vias: 79.12,47.63
N$471  (via drill 0.89 pad 1.65)
  other vias: 81.66,50.17
N$472  (via drill 0.89 pad 1.65)
  other vias: 81.66,47.63
N$473  (via drill 0.89 pad 1.65)
  other vias: 84.2,50.17
N$474  (via drill 0.89 pad 1.65)
  other vias: 84.2,47.63
N$475  (via drill 0.89 pad 1.65)
  other vias: 86.74,47.63
N$476  (via drill 0.89 pad 1.65)
  other vias: 89.28,47.63
N$477  (via drill 0.89 pad 1.65)
  other vias: 91.82,47.63
N$478  (via drill 0.89 pad 1.65)
  other vias: 94.36,47.63
N$479  (via drill 0.89 pad 1.65)
  other vias: 96.9,47.63
N$480  (via drill 0.89 pad 1.65)
  other vias: 99.44,47.63
N$481  (via drill 0.89 pad 1.65)
  other vias: 101.98,47.63
N$482  (via drill 0.89 pad 1.65)
  other vias: 104.52,47.63
N$483  (via drill 0.89 pad 1.65)
  other vias: 86.74,50.17
N$484  (via drill 0.89 pad 1.65)
  other vias: 89.28,50.17
N$485  (via drill 0.89 pad 1.65)
  other vias: 91.82,50.17
N$486  (via drill 0.89 pad 1.65)
  other vias: 94.36,50.17
N$487  (via drill 0.89 pad 1.65)
  other vias: 96.9,50.17
N$488  (via drill 0.89 pad 1.65)
  other vias: 99.44,50.17
N$489  (via drill 0.89 pad 1.65)
  other vias: 101.98,50.17
N$490  (via drill 0.89 pad 1.65)
  other vias: 104.52,50.17
N$491  (via drill 0.89 pad 1.65)
  other vias: 41.02,52.71
N$492  (via drill 0.89 pad 1.65)
  other vias: 43.56,52.71
N$493  (via drill 0.89 pad 1.65)
  other vias: 46.1,52.71
N$494  (via drill 0.89 pad 1.65)
  other vias: 48.64,52.71
N$495  (via drill 0.89 pad 1.65)
  other vias: 51.18,52.71
N$496  (via drill 0.89 pad 1.65)
  other vias: 41.02,55.25
N$497  (via drill 0.89 pad 1.65)
  other vias: 43.56,55.25
N$498  (via drill 0.89 pad 1.65)
  other vias: 46.1,55.25
N$499  (via drill 0.89 pad 1.65)
  other vias: 48.64,55.25
N$500  (via drill 0.89 pad 1.65)
  other vias: 51.18,55.25
N$501  (via drill 0.89 pad 1.65)
  other vias: 53.72,52.71
N$502  (via drill 0.89 pad 1.65)
  other vias: 53.72,55.25
N$503  (via drill 0.89 pad 1.65)
  other vias: 56.26,55.25
N$504  (via drill 0.89 pad 1.65)
  other vias: 56.26,52.71
N$505  (via drill 0.89 pad 1.65)
  other vias: 58.8,55.25
N$506  (via drill 0.89 pad 1.65)
  other vias: 58.8,52.71
N$507  (via drill 0.89 pad 1.65)
  other vias: 61.34,78.11
N$508  (via drill 0.89 pad 1.65)
  other vias: 61.34,55.25
N$509  (via drill 0.89 pad 1.65)
  other vias: 66.42,52.71
N$510  (via drill 0.89 pad 1.65)
  other vias: 68.96,55.25
N$511  (via drill 0.89 pad 1.65)
  other vias: 68.96,52.71
N$512  (via drill 0.89 pad 1.65)
  other vias: 71.5,55.25
N$513  (via drill 0.89 pad 1.65)
  other vias: 71.5,52.71
N$514  (via drill 0.89 pad 1.65)
  other vias: 74.04,55.25
N$515  (via drill 0.89 pad 1.65)
  other vias: 74.04,52.71
N$516  (via drill 0.89 pad 1.65)
  other vias: 76.58,55.25
N$517  (via drill 0.89 pad 1.65)
  other vias: 76.58,52.71
N$518  (via drill 0.89 pad 1.65)
  other vias: 79.12,55.25
N$519  (via drill 0.89 pad 1.65)
  other vias: 79.12,52.71
N$520  (via drill 0.89 pad 1.65)
  other vias: 81.66,55.25
N$521  (via drill 0.89 pad 1.65)
  other vias: 81.66,52.71
N$522  (via drill 0.89 pad 1.65)
  other vias: 84.2,55.25
N$523  (via drill 0.89 pad 1.65)
  other vias: 84.2,52.71
N$524  (via drill 0.89 pad 1.65)
  other vias: 86.74,52.71
N$525  (via drill 0.89 pad 1.65)
  other vias: 89.28,52.71
N$526  (via drill 0.89 pad 1.65)
  other vias: 91.82,52.71
N$527  (via drill 0.89 pad 1.65)
  other vias: 94.36,52.71
N$528  (via drill 0.89 pad 1.65)
  other vias: 96.9,52.71
N$529  (via drill 0.89 pad 1.65)
  other vias: 99.44,52.71
N$530  (via drill 0.89 pad 1.65)
  other vias: 101.98,52.71
N$531  (via drill 0.89 pad 1.65)
  other vias: 104.52,52.71
N$532  (via drill 0.89 pad 1.65)
  other vias: 86.74,55.25
N$533  (via drill 0.89 pad 1.65)
  other vias: 89.28,55.25
N$534  (via drill 0.89 pad 1.65)
  other vias: 91.82,55.25
N$535  (via drill 0.89 pad 1.65)
  other vias: 94.36,55.25
N$536  (via drill 0.89 pad 1.65)
  other vias: 96.9,55.25
N$537  (via drill 0.89 pad 1.65)
  other vias: 99.44,55.25
N$538  (via drill 0.89 pad 1.65)
  other vias: 101.98,55.25
N$539  (via drill 0.89 pad 1.65)
  other vias: 104.52,55.25
N$540  (via drill 0.89 pad 1.65)
  other vias: 41.02,57.79
N$541  (via drill 0.89 pad 1.65)
  other vias: 43.56,57.79
N$542  (via drill 0.89 pad 1.65)
  other vias: 46.1,57.79
N$543  (via drill 0.89 pad 1.65)
  other vias: 48.64,57.79
N$544  (via drill 0.89 pad 1.65)
  other vias: 51.18,57.79
N$545  (via drill 0.89 pad 1.65)
  Top 0.406: v41.02,60.33 41.02,52.71
N$546  (via drill 0.89 pad 1.65)
  other vias: 43.56,60.33
N$547  (via drill 0.89 pad 1.65)
  other vias: 46.1,60.33
N$548  (via drill 0.89 pad 1.65)
  other vias: 48.64,60.33
N$549  (via drill 0.89 pad 1.65)
  other vias: 51.18,60.33
N$550  (via drill 0.89 pad 1.65)
  other vias: 53.72,57.79
N$551  (via drill 0.89 pad 1.65)
  other vias: 53.72,60.33
N$552  (via drill 0.89 pad 1.65)
  other vias: 56.26,60.33
N$553  (via drill 0.89 pad 1.65)
  other vias: 56.26,57.79
N$554  (via drill 0.89 pad 1.65)
  other vias: 58.8,60.33
N$555  (via drill 0.89 pad 1.65)
  other vias: 58.8,57.79
N$556  (via drill 0.89 pad 1.65)
  other vias: 61.34,57.79
N$557  (via drill 0.89 pad 1.65)
  other vias: 61.34,60.33
N$558  (via drill 0.89 pad 1.65)
  other vias: 66.42,57.79
N$559  (via drill 0.89 pad 1.65)
  other vias: 68.96,60.33
N$560  (via drill 0.89 pad 1.65)
  other vias: 68.96,57.79
N$561  (via drill 0.89 pad 1.65)
  other vias: 71.5,60.33
N$562  (via drill 0.89 pad 1.65)
  other vias: 71.5,57.79
N$563  (via drill 0.89 pad 1.65)
  other vias: 74.04,60.33
N$564  (via drill 0.89 pad 1.65)
  other vias: 74.04,57.79
N$565  (via drill 0.89 pad 1.65)
  other vias: 76.58,60.33
N$566  (via drill 0.89 pad 1.65)
  other vias: 76.58,57.79
N$567  (via drill 0.89 pad 1.65)
  other vias: 79.12,60.33
N$568  (via drill 0.89 pad 1.65)
  other vias: 79.12,57.79
N$569  (via drill 0.89 pad 1.65)
  other vias: 81.66,60.33
N$570  (via drill 0.89 pad 1.65)
  other vias: 81.66,57.79
N$571  (via drill 0.89 pad 1.65)
  other vias: 84.2,60.33
N$572  (via drill 0.89 pad 1.65)
  other vias: 84.2,57.79
N$573  (via drill 0.89 pad 1.65)
  other vias: 86.74,57.79
N$574  (via drill 0.89 pad 1.65)
  other vias: 89.28,57.79
N$575  (via drill 0.89 pad 1.65)
  other vias: 91.82,57.79
N$576  (via drill 0.89 pad 1.65)
  other vias: 94.36,57.79
N$577  (via drill 0.89 pad 1.65)
  other vias: 96.9,57.79
N$578  (via drill 0.89 pad 1.65)
  other vias: 99.44,57.79
N$579  (via drill 0.89 pad 1.65)
  other vias: 101.98,57.79
N$580  (via drill 0.89 pad 1.65)
  other vias: 104.52,57.79
N$581  (via drill 0.89 pad 1.65)
  other vias: 86.74,60.33
N$582  (via drill 0.89 pad 1.65)
  other vias: 89.28,60.33
N$583  (via drill 0.89 pad 1.65)
  other vias: 91.82,60.33
N$584  (via drill 0.89 pad 1.65)
  other vias: 94.36,60.33
N$585  (via drill 0.89 pad 1.65)
  other vias: 96.9,60.33
N$586  (via drill 0.89 pad 1.65)
  other vias: 99.44,60.33
N$587  (via drill 0.89 pad 1.65)
  other vias: 101.98,60.33
N$588  (via drill 0.89 pad 1.65)
  other vias: 104.52,60.33
N$589  (via drill 0.89 pad 1.65)
  other vias: 41.02,62.87
N$590  (via drill 0.89 pad 1.65)
  other vias: 43.56,62.87
N$591  (via drill 0.89 pad 1.65)
  other vias: 46.1,62.87
N$592  (via drill 0.89 pad 1.65)
  other vias: 48.64,62.87
N$593  (via drill 0.89 pad 1.65)
  other vias: 51.18,62.87
N$594  (via drill 0.89 pad 1.65)
  other vias: 41.02,65.41
N$595  (via drill 0.89 pad 1.65)
  other vias: 43.56,65.41
N$596  (via drill 0.89 pad 1.65)
  other vias: 46.1,65.41
N$597  (via drill 0.89 pad 1.65)
  other vias: 48.64,65.41
N$598  (via drill 0.89 pad 1.65)
  other vias: 51.18,65.41
N$599  (via drill 0.89 pad 1.65)
  other vias: 53.72,62.87
N$600  (via drill 0.89 pad 1.65)
  other vias: 53.72,65.41
N$601  (via drill 0.89 pad 1.65)
  other vias: 56.26,65.41
N$602  (via drill 0.89 pad 1.65)
  other vias: 56.26,62.87
N$603  (via drill 0.89 pad 1.65)
  other vias: 58.8,65.41
N$604  (via drill 0.89 pad 1.65)
  other vias: 58.8,62.87
N$605  (via drill 0.89 pad 1.65)
  other vias: 63.88,78.11
N$606  (via drill 0.89 pad 1.65)
  other vias: 61.34,65.41
N$607  (via drill 0.89 pad 1.65)
  other vias: 66.42,62.87
N$608  (via drill 0.89 pad 1.65)
  other vias: 68.96,65.41
N$609  (via drill 0.89 pad 1.65)
  other vias: 68.96,62.87
N$610  (via drill 0.89 pad 1.65)
  other vias: 71.5,65.41
N$611  (via drill 0.89 pad 1.65)
  other vias: 71.5,62.87
N$612  (via drill 0.89 pad 1.65)
  other vias: 74.04,65.41
N$613  (via drill 0.89 pad 1.65)
  other vias: 74.04,62.87
N$614  (via drill 0.89 pad 1.65)
  other vias: 76.58,65.41
N$615  (via drill 0.89 pad 1.65)
  other vias: 76.58,62.87
N$616  (via drill 0.89 pad 1.65)
  other vias: 79.12,65.41
N$617  (via drill 0.89 pad 1.65)
  other vias: 79.12,62.87
N$618  (via drill 0.89 pad 1.65)
  other vias: 81.66,65.41
N$619  (via drill 0.89 pad 1.65)
  other vias: 81.66,62.87
N$620  (via drill 0.89 pad 1.65)
  other vias: 84.2,65.41
N$621  (via drill 0.89 pad 1.65)
  other vias: 84.2,62.87
N$622  (via drill 0.89 pad 1.65)
  other vias: 86.74,62.87
N$623  (via drill 0.89 pad 1.65)
  other vias: 89.28,62.87
N$624  (via drill 0.89 pad 1.65)
  other vias: 91.82,62.87
N$625  (via drill 0.89 pad 1.65)
  other vias: 94.36,62.87
N$626  (via drill 0.89 pad 1.65)
  other vias: 96.9,62.87
N$627  (via drill 0.89 pad 1.65)
  other vias: 99.44,62.87
N$628  (via drill 0.89 pad 1.65)
  other vias: 101.98,62.87
N$629  (via drill 0.89 pad 1.65)
  other vias: 104.52,62.87
N$630  (via drill 0.89 pad 1.65)
  other vias: 86.74,65.41
N$631  (via drill 0.89 pad 1.65)
  other vias: 89.28,65.41
N$632  (via drill 0.89 pad 1.65)
  other vias: 91.82,65.41
N$633  (via drill 0.89 pad 1.65)
  other vias: 94.36,65.41
N$634  (via drill 0.89 pad 1.65)
  other vias: 96.9,65.41
N$635  (via drill 0.89 pad 1.65)
  other vias: 99.44,65.41
N$636  (via drill 0.89 pad 1.65)
  other vias: 101.98,65.41
N$637  (via drill 0.89 pad 1.65)
  other vias: 104.52,65.41
N$638  (via drill 0.89 pad 1.65)
  other vias: 41.02,67.95
N$639  (via drill 0.89 pad 1.65)
  other vias: 43.56,67.95
N$640  (via drill 0.89 pad 1.65)
  other vias: 46.1,67.95
N$641  (via drill 0.89 pad 1.65)
  other vias: 48.64,67.95
N$642  (via drill 0.89 pad 1.65)
  other vias: 51.18,67.95
N$643  (via drill 0.89 pad 1.65)
  Top 0.406: v41.02,70.49 41.02,62.87
N$644  (via drill 0.89 pad 1.65)
  other vias: 43.56,70.49
N$645  (via drill 0.89 pad 1.65)
  other vias: 46.1,70.49
N$646  (via drill 0.89 pad 1.65)
  other vias: 48.64,70.49
N$647  (via drill 0.89 pad 1.65)
  other vias: 51.18,70.49
N$648  (via drill 0.89 pad 1.65)
  other vias: 53.72,67.95
N$649  (via drill 0.89 pad 1.65)
  other vias: 53.72,70.49
N$650  (via drill 0.89 pad 1.65)
  other vias: 56.26,70.49
N$651  (via drill 0.89 pad 1.65)
  other vias: 56.26,67.95
N$652  (via drill 0.89 pad 1.65)
  other vias: 58.8,70.49
N$653  (via drill 0.89 pad 1.65)
  other vias: 58.8,67.95
N$654  (via drill 0.89 pad 1.65)
  other vias: 63.88,75.57
N$655  (via drill 0.89 pad 1.65)
  other vias: 61.34,70.49
N$656  (via drill 0.89 pad 1.65)
  other vias: 66.42,67.95
N$657  (via drill 0.89 pad 1.65)
  other vias: 68.96,70.49
N$658  (via drill 0.89 pad 1.65)
  other vias: 68.96,67.95
N$659  (via drill 0.89 pad 1.65)
  other vias: 71.5,70.49
N$660  (via drill 0.89 pad 1.65)
  other vias: 71.5,67.95
N$661  (via drill 0.89 pad 1.65)
  other vias: 74.04,70.49
N$662  (via drill 0.89 pad 1.65)
  other vias: 74.04,67.95
N$663  (via drill 0.89 pad 1.65)
  other vias: 76.58,70.49
N$664  (via drill 0.89 pad 1.65)
  other vias: 76.58,67.95
N$665  (via drill 0.89 pad 1.65)
  other vias: 79.12,70.49
N$666  (via drill 0.89 pad 1.65)
  other vias: 79.12,67.95
N$667  (via drill 0.89 pad 1.65)
  other vias: 81.66,70.49
N$668  (via drill 0.89 pad 1.65)
  other vias: 81.66,67.95
N$669  (via drill 0.89 pad 1.65)
  other vias: 84.2,70.49
N$670  (via drill 0.89 pad 1.65)
  other vias: 84.2,67.95
N$671  (via drill 0.89 pad 1.65)
  other vias: 86.74,67.95
N$672  (via drill 0.89 pad 1.65)
  other vias: 89.28,67.95
N$673  (via drill 0.89 pad 1.65)
  other vias: 91.82,67.95
N$674  (via drill 0.89 pad 1.65)
  other vias: 94.36,67.95
N$675  (via drill 0.89 pad 1.65)
  other vias: 96.9,67.95
N$676  (via drill 0.89 pad 1.65)
  other vias: 99.44,67.95
N$677  (via drill 0.89 pad 1.65)
  other vias: 101.98,67.95
N$678  (via drill 0.89 pad 1.65)
  other vias: 104.52,67.95
N$679  (via drill 0.89 pad 1.65)
  other vias: 86.74,70.49
N$680  (via drill 0.89 pad 1.65)
  other vias: 89.28,70.49
N$681  (via drill 0.89 pad 1.65)
  other vias: 91.82,70.49
N$682  (via drill 0.89 pad 1.65)
  other vias: 94.36,70.49
N$683  (via drill 0.89 pad 1.65)
  other vias: 96.9,70.49
N$684  (via drill 0.89 pad 1.65)
  other vias: 99.44,70.49
N$685  (via drill 0.89 pad 1.65)
  other vias: 101.98,70.49
N$686  (via drill 0.89 pad 1.65)
  other vias: 104.52,70.49
N$687  (via drill 0.89 pad 1.65)
  other vias: 41.02,73.03
N$688  (via drill 0.89 pad 1.65)
  other vias: 43.56,73.03
N$689  (via drill 0.89 pad 1.65)
  other vias: 46.1,73.03
N$690  (via drill 0.89 pad 1.65)
  other vias: 48.64,73.03
N$691  (via drill 0.89 pad 1.65)
  other vias: 51.18,73.03
N$692  (via drill 0.89 pad 1.65)
  other vias: 41.02,75.57
N$693  (via drill 0.89 pad 1.65)
  other vias: 43.56,75.57
N$694  (via drill 0.89 pad 1.65)
  other vias: 46.1,75.57
N$695  (via drill 0.89 pad 1.65)
  other vias: 48.64,75.57
N$696  (via drill 0.89 pad 1.65)
  other vias: 51.18,75.57
N$697  (via drill 0.89 pad 1.65)
  other vias: 53.72,73.03
N$698  (via drill 0.89 pad 1.65)
  other vias: 53.72,75.57
N$699  (via drill 0.89 pad 1.65)
  other vias: 56.26,75.57
N$700  (via drill 0.89 pad 1.65)
  other vias: 56.26,73.03
N$701  (via drill 0.89 pad 1.65)
  other vias: 58.8,75.57
N$702  (via drill 0.89 pad 1.65)
  other vias: 58.8,73.03
N$703  (via drill 0.89 pad 1.65)
  other vias: 66.42,75.57
N$704  (via drill 0.89 pad 1.65)
  other vias: 61.34,75.57
N$705  (via drill 0.89 pad 1.65)
  other vias: 66.42,73.03
N$706  (via drill 0.89 pad 1.65)
  other vias: 68.96,75.57
N$707  (via drill 0.89 pad 1.65)
  other vias: 68.96,73.03
N$708  (via drill 0.89 pad 1.65)
  other vias: 71.5,75.57
N$709  (via drill 0.89 pad 1.65)
  other vias: 71.5,73.03
N$710  (via drill 0.89 pad 1.65)
  other vias: 74.04,75.57
N$711  (via drill 0.89 pad 1.65)
  other vias: 74.04,73.03
N$712  (via drill 0.89 pad 1.65)
  other vias: 76.58,75.57
N$713  (via drill 0.89 pad 1.65)
  other vias: 76.58,73.03
N$714  (via drill 0.89 pad 1.65)
  other vias: 79.12,75.57
N$715  (via drill 0.89 pad 1.65)
  other vias: 79.12,73.03
N$716  (via drill 0.89 pad 1.65)
  other vias: 81.66,75.57
N$717  (via drill 0.89 pad 1.65)
  other vias: 81.66,73.03
N$718  (via drill 0.89 pad 1.65)
  other vias: 84.2,75.57
N$719  (via drill 0.89 pad 1.65)
  other vias: 84.2,73.03
N$720  (via drill 0.89 pad 1.65)
  other vias: 86.74,73.03
N$721  (via drill 0.89 pad 1.65)
  other vias: 89.28,73.03
N$722  (via drill 0.89 pad 1.65)
  other vias: 91.82,73.03
N$723  (via drill 0.89 pad 1.65)
  other vias: 94.36,73.03
N$724  (via drill 0.89 pad 1.65)
  other vias: 96.9,73.03
N$725  (via drill 0.89 pad 1.65)
  other vias: 99.44,73.03
N$726  (via drill 0.89 pad 1.65)
  other vias: 101.98,73.03
N$727  (via drill 0.89 pad 1.65)
  other vias: 104.52,73.03
N$728  (via drill 0.89 pad 1.65)
  other vias: 86.74,75.57
N$729  (via drill 0.89 pad 1.65)
  other vias: 89.28,75.57
N$730  (via drill 0.89 pad 1.65)
  other vias: 91.82,75.57
N$731  (via drill 0.89 pad 1.65)
  other vias: 94.36,75.57
N$732  (via drill 0.89 pad 1.65)
  other vias: 96.9,75.57
N$733  (via drill 0.89 pad 1.65)
  other vias: 99.44,75.57
N$734  (via drill 0.89 pad 1.65)
  other vias: 101.98,75.57
N$735  (via drill 0.89 pad 1.65)
  other vias: 104.52,75.57
N$736  (via drill 0.89 pad 1.65)
  other vias: 41.02,78.11
N$737  (via drill 0.89 pad 1.65)
  other vias: 43.56,78.11
N$738  (via drill 0.89 pad 1.65)
  other vias: 46.1,78.11
N$739  (via drill 0.89 pad 1.65)
  other vias: 48.64,78.11
N$740  (via drill 0.89 pad 1.65)
  other vias: 51.18,78.11
N$741  (via drill 0.89 pad 1.65)
  other vias: 61.34,73.03
N$742  (via drill 0.89 pad 1.65)
  other vias: 43.56,80.65
N$743  (via drill 0.89 pad 1.65)
  other vias: 46.1,80.65
N$744  (via drill 0.89 pad 1.65)
  other vias: 48.64,80.65
N$745  (via drill 0.89 pad 1.65)
  other vias: 51.18,80.65
N$746  (via drill 0.89 pad 1.65)
  other vias: 53.72,78.11
N$747  (via drill 0.89 pad 1.65)
  other vias: 53.72,80.65
N$748  (via drill 0.89 pad 1.65)
  other vias: 56.26,80.65
N$749  (via drill 0.89 pad 1.65)
  other vias: 56.26,78.11
N$750  (via drill 0.89 pad 1.65)
  other vias: 58.8,80.65
N$751  (via drill 0.89 pad 1.65)
  other vias: 58.8,78.11
N$753  (via drill 0.89 pad 1.65)
  other vias: 61.34,80.65
N$754  (via drill 0.89 pad 1.65)
  other vias: 66.42,78.11
N$755  (via drill 0.89 pad 1.65)
  other vias: 68.96,80.65
N$756  (via drill 0.89 pad 1.65)
  other vias: 68.96,78.11
N$757  (via drill 0.89 pad 1.65)
  other vias: 71.5,80.65
N$758  (via drill 0.89 pad 1.65)
  other vias: 71.5,78.11
N$759  (via drill 0.89 pad 1.65)
  other vias: 74.04,80.65
N$760  (via drill 0.89 pad 1.65)
  other vias: 74.04,78.11
N$761  (via drill 0.89 pad 1.65)
  other vias: 76.58,80.65
N$762  (via drill 0.89 pad 1.65)
  other vias: 76.58,78.11
N$763  (via drill 0.89 pad 1.65)
  other vias: 79.12,80.65
N$764  (via drill 0.89 pad 1.65)
  other vias: 79.12,78.11
N$765  (via drill 0.89 pad 1.65)
  other vias: 81.66,80.65
N$766  (via drill 0.89 pad 1.65)
  other vias: 81.66,78.11
N$767  (via drill 0.89 pad 1.65)
  other vias: 84.2,80.65
N$768  (via drill 0.89 pad 1.65)
  other vias: 84.2,78.11
N$769  (via drill 0.89 pad 1.65)
  other vias: 86.74,78.11
N$770  (via drill 0.89 pad 1.65)
  other vias: 89.28,78.11
N$771  (via drill 0.89 pad 1.65)
  other vias: 91.82,78.11
N$772  (via drill 0.89 pad 1.65)
  other vias: 94.36,78.11
N$773  (via drill 0.89 pad 1.65)
  other vias: 96.9,78.11
N$774  (via drill 0.89 pad 1.65)
  other vias: 99.44,78.11
N$775  (via drill 0.89 pad 1.65)
  other vias: 101.98,78.11
N$776  (via drill 0.89 pad 1.65)
  other vias: 104.52,78.11
N$777  (via drill 0.89 pad 1.65)
  other vias: 86.74,80.65
N$778  (via drill 0.89 pad 1.65)
  other vias: 89.28,80.65
N$779  (via drill 0.89 pad 1.65)
  other vias: 91.82,80.65
N$780  (via drill 0.89 pad 1.65)
  other vias: 94.36,80.65
N$781  (via drill 0.89 pad 1.65)
  other vias: 96.9,80.65
N$782  (via drill 0.89 pad 1.65)
  other vias: 99.44,80.65
N$783  (via drill 0.89 pad 1.65)
  other vias: 101.98,80.65
N$784  (via drill 0.89 pad 1.65)
  other vias: 104.52,80.65
N$785  (via drill 0.89 pad 1.65)
  other vias: 63.88,73.03
N$786  (via drill 0.89 pad 1.65)
  other vias: 63.88,70.49
N$787  (via drill 0.89 pad 1.65)
  Top 0.406: v41.02,80.65 41.02,73.03
N$788  (via drill 0.89 pad 1.65)
  other vias: 66.42,70.49
N$789  (via drill 0.89 pad 1.65)
  other vias: 63.88,67.95
N$790  (via drill 0.89 pad 1.65)
  other vias: 61.34,67.95
N$791  (via drill 0.89 pad 1.65)
  other vias: 63.88,65.41
N$792  (via drill 0.89 pad 1.65)
  other vias: 66.42,65.41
